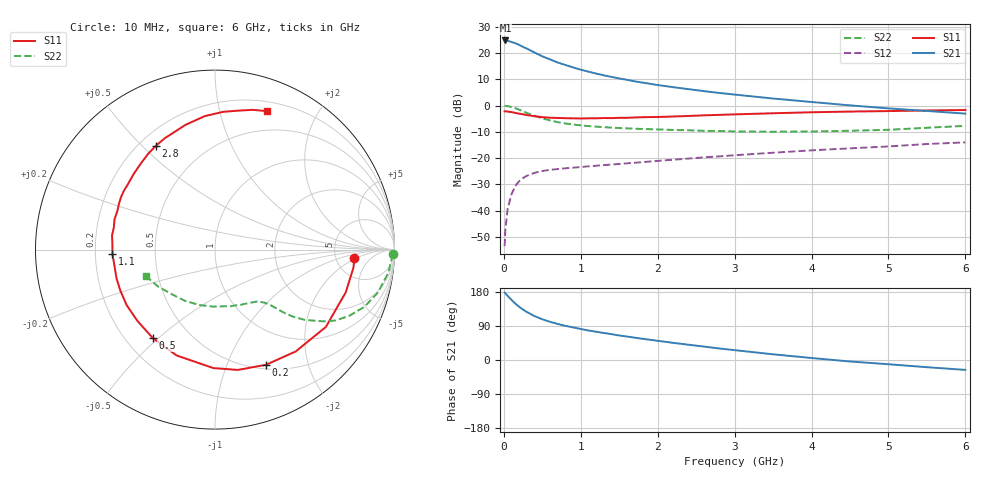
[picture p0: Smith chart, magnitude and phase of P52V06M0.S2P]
! SIEMENS Small Signal Semiconductors
! BFP183
! Si NPN RF Bipolar Junction Transistor in SOT143
! VCE = 2 V  IC = 6 mA
! Common Emitter S-Parameters:  March  1996
# GHz  S  MA  R  50
!  f  S11  S21  S12  S22
! GHz  MAG  ANG  MAG  ANG  MAG  ANG  MAG  ANG
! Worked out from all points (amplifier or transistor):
!   36 points, 10 MHz to 6 GHz, reference 50 ohm
!   highest |S21| = 24.8 dB at 20 MHz (marker M1)
!   |S21| within 3 dB of that: start of sweep to 291.1 MHz
!   unconditionally stable (mu >= 1): 1.414 GHz to 5.623 GHz
!   at 250 MHz: K = 0.23, MSG = 25.0 dB, |S12| = -27.6 dB
!   at 1.4 GHz: K = 1.00, MSG = 16.7 dB, |S12| = -22.5 dB
!   at 6 GHz: K = 0.96, MSG = 5.5 dB, |S12| = -14.0 dB
!   lowest NFmin = 1.20 dB at 450 MHz
!   S11 on the Smith chart (normalised r, x): 10 MHz: 7.62, -1.73; 200 MHz: 0.55, -1.39; 500 MHz: 0.31, -0.48; 1.1 GHz: 0.27, -0.02; 2.8 GHz: 0.27, +0.55; 6 GHz: 0.29, +1.40
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0.01  0.7784 -3.3  17.2 177.9  0.0021 83.0  0.9916 -1.5
0.02  0.7777 -7.5  17.4 176.0  0.0044 84.4  0.9852 -3.1
0.05  0.7664 -18.1  17.13 169.0  0.0109 82.8  0.9751 -7.5
0.1  0.7532 -34.9  16.26 158.6  0.0206 71.3  0.9389 -14.7
0.15  0.7241 -51.6  15.46 148.7  0.0295 64.5  0.8912 -21.0
0.2  0.7018 -66.1  14.31 140.3  0.0365 59.0  0.8354 -26.1
0.25  0.6825 -79.2  13.12 132.8  0.0417 53.8  0.7804 -30.4
0.3  0.6601 -90.8  12.15 126.6  0.0461 49.3  0.7245 -33.5
0.4  0.6274 -110.0  10.23 115.7  0.0524 43.5  0.6367 -38.0
0.5  0.6021 -125.3  8.665 107.5  0.0567 39.0  0.5723 -40.7
0.6  0.587 -137.5  7.588 100.8  0.0598 36.5  0.5219 -42.4
0.7  0.5813 -147.8  6.611 95.2  0.0618 35.0  0.484 -43.5
0.9  0.5716 -163.7  5.331 86.1  0.0657 33.4  0.4359 -45.1
1.1  0.5718 -177.5  4.43 77.9  0.0698 33.0  0.4069 -46.8
1.5  0.5847 163.3  3.291 64.7  0.0772 33.5  0.373 -51.0
1.8  0.6001 150.7  2.745 56.1  0.0838 34.1  0.3587 -55.2
2.2  0.6194 136.8  2.242 45.3  0.093 34.4  0.3434 -62.0
2.8  0.6657 119.6  1.742 30.4  0.1079 33.6  0.3276 -74.4
3.5  0.7139 103.4  1.362 15.0  0.1265 31.7  0.3178 -91.7
4.5  0.7692 86.5  1.01 -3.9  0.1533 26.4  0.3314 -120.9
5.5  0.8066 74.9  0.79 -19.0  0.1853 20.8  0.3779 -147.0
6  0.8236 69.5  0.703 -26.1  0.1992 16.7  0.4111 -158.7
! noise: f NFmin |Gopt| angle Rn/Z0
0.45  1.2  0.21  41  0.24
0.9  1.25  0.24  101  0.21
1.8  2  0.32  175  0.14
